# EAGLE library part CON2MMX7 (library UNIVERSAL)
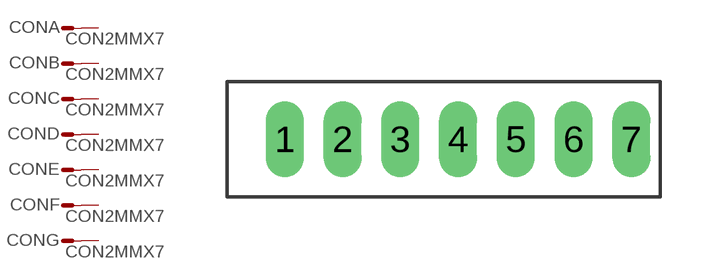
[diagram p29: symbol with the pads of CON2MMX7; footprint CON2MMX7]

Designator prefix CON; gates A=CONPIN B=CONPIN C=CONPIN D=CONPIN E=CONPIN F=CONPIN G=CONPIN

## CON2MMX7  [CON2MMX7]
1  A:S  pas
2  B:S  pas
3  C:S  pas
4  D:S  pas
5  E:S  pas
6  F:S  pas
7  G:S  pas

## Footprint CON2MMX7 (pad centres in mm)
drill 0.8 pad 1.016 long: 1 0,0; 2 2,0; 3 4,0; 4 6,0; 5 8,0; 6 10,0; 7 12,0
